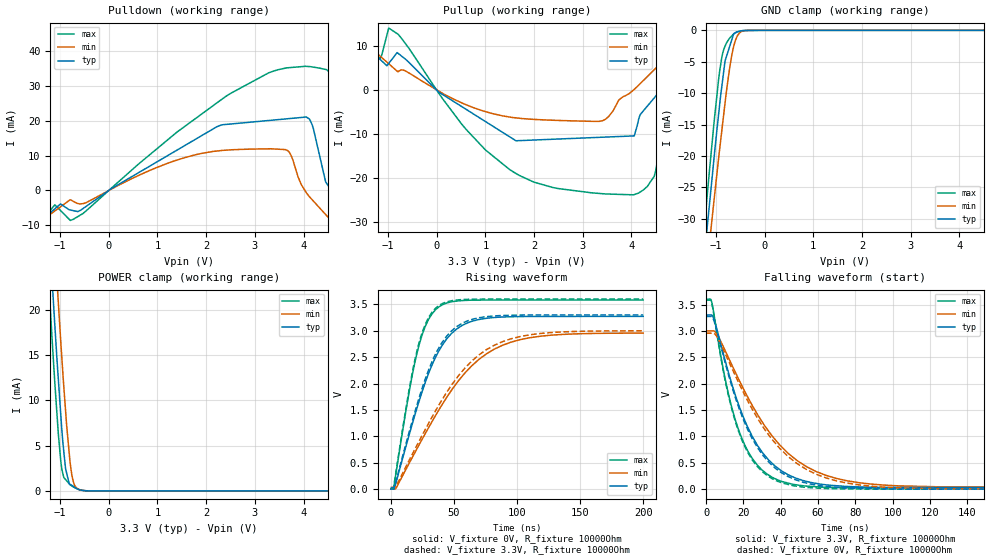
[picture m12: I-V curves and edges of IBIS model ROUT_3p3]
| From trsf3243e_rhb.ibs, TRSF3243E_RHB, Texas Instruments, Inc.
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[Model]   ROUT_3p3
Model_type   3-state
Polarity   Non-Inverting
Vmeas = 1.65
Vref = 0
Cref = 150pF
Rref = 3000
|variable   typ   min   max
C_comp   1.47pF   1.38pF   1.52pF
|C_pullup   1.38pF   1.27pF   1.45pF
|C_pulldown   1.80pF   1.75pF   1.86pF
[Voltage Range]   3.3   3   3.6
[Temperature Range]   27   110   -40
[Pullup Reference]   3.3   3   3.6
[Pulldown Reference]   0   0   0
[Power Clamp Reference]   3.3   3   3.6
[GND Clamp Reference]   0   0   0
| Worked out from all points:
|   slope of the pulldown table from 0 to 0.495 V, typ, clamps not added: 119 ohm
|   slope of the pullup table from 0 to 0.495 V, typ, clamps not added: 136 ohm
|   GND clamp passes 1 mA (typ) near -0.65 V on its own axis
|   POWER clamp passes 1 mA (typ) near -0.82 V on its own axis
|   falling waveform, V_fixture 3.3V, R_fixture 10000Ohm: 20-80 % time 21.7ns typ, 32.6ns min, 15.9ns max; typ from 3.3 V to 0.029 V
|   rising waveform, V_fixture 0V, R_fixture 10000Ohm: 20-80 % time 27.9ns typ, 48.7ns min, 17.3ns max; typ from 0 V to 3.27 V
|   rising waveform, V_fixture 3.3V, R_fixture 10000Ohm: 20-80 % time 27.3ns typ, 47.1ns min, 17ns max; typ from 0.029 V to 3.3 V
|   falling waveform, V_fixture 0V, R_fixture 10000Ohm: 20-80 % time 21.6ns typ, 32.1ns min, 15.9ns max; typ from 3.27 V to 0 V
[Pulldown]
|   Voltage   I(typ)   I(min)   I(max)
-3.3V     -787.1uA   -298.2uA   -879.3uA
-3.13V    -9.259mA   -8.11mA    -9.971mA
-788.7mV  -5.612mA   -2.71mA    -8.598mA
2.735V    19.39mA    11.81mA    29.64mA
4.042V    21.08mA    -312.1uA   35.66mA
4.523V    1.033mA    -7.969mA   33.99mA
4.925V    -7.207mA   -9.102mA   4.57mA
5.433V    -7.855mA   -9.28mA    -8.328mA
6.366V    -7.517mA   -9.606mA   -7.618mA
6.522V    -7.461mA   -6.718mA   -2.416mA
6.532V    24.7mA     -6.523mA   24.29mA
6.6V      231.2mA    268.8mA    195.7mA
[GND Clamp]
|   Voltage   I(typ)   I(min)   I(max)
-3.3V     -210.1mA   -202.3mA   -218.6mA
-1.348V   -45.17mA   -50.25mA   -41.18mA
-1.208V   -33.83mA   -39.74mA   -28.91mA
-1.175V   -31.12mA   -37.23mA   -26.05mA
-1.107V   -25.78mA   -32.11mA   -20.34mA
-942mV    -13.28mA   -20.29mA   -7.725mA
-879.8mV  -9.08mA    -16.12mA   -4.389mA
-811.2mV  -4.875mA   -11.57mA   -2.536mA
-686.3mV  -1.833mA   -4.566mA   -987.9uA
-577mV    -278.2uA   -1.197mA   -309.3uA
-315.2mV  -33.26uA   -7.242uA   -7.414uA
6.6V      0A         0A         0A
[Pullup]
|   Voltage   I(typ)   I(min)   I(max)
-3.3V     131.1uA    87.96uA    178.1uA
-3.13V    9.92mA     9.846mA    9.995mA
-1.163V   7.022mA    7.761mA    7.124mA
-984.1mV  6.064mA    6.007mA    14.15mA
1.499V    -10.66mA   -6.155mA   -18.13mA
3.404V    -10.76mA   -7.017mA   -23.64mA
4.042V    -10.46mA   18.97uA    -23.9mA
5.433V    5.648mA    6.097mA    6.407mA
6.366V    4.745mA    6.255mA    5.441mA
6.52V     4.596mA    3.972mA    5.281mA
6.532V    -24.61mA   3.786mA    -25.75mA
6.6V      -212.1mA   -227.5mA   -193.1mA
[POWER Clamp]
|   Voltage   I(typ)   I(min)   I(max)
-3.3V     230.9mA    239.1mA    225mA
-1.254V   31.57mA    40.43mA    25.24mA
-1.175V   24.31mA    33.19mA    17.85mA
-1.131V   20.41mA    29.18mA    13.95mA
-1.06V    14.27mA    22.94mA    8.245mA
-1.035V   12.33mA    20.8mA     6.311mA
-961.9mV  6.695mA    14.63mA    2.369mA
-887.3mV  2.484mA    8.947mA    1.267mA
-795.8mV  739.7uA    3.272mA    699uA
-760mV    616.4uA    1.855mA    553.7uA
-633.3mV  180.3uA    217uA      201.5uA
6.6V      0A         0A         0A
[Ramp]
R_load = 10000
|   typ   min   max
dV/dt_r   1.96363/2.79356e-08   1.77363/4.8671e-08   2.14915/1.72734e-08
dV/dt_f   1.96255/2.17589e-08   1.77823/3.26253e-08   2.14523/1.59509e-08
[Falling Waveform]
V_fixture = 3.3V
V_fixture_min = 3V
V_fixture_max = 3.6V
R_fixture = 10000Ohm
C_fixture = 0F
|   Time   V(typ)   V(min)   V(max)
0s        3.3V       3V         3.6V
3.021ns   3.301V     3.001V     3.545V
5.942ns   3.011V     2.932V     2.932V
11.03ns   2.329V     2.563V     1.951V
17.15ns   1.628V     2.106V     1.149V
24.77ns   996.4mV    1.584V     580.2mV
35.47ns   486.9mV    1.005V     223.6mV
53.77ns   147.3mV    427.5mV    58.24mV
75.54ns   51.26mV    158.8mV    29.98mV
200ns     29.08mV    36.28mV    24.61mV
[Rising Waveform]
V_fixture = 0V
V_fixture_min = 0V
V_fixture_max = 0V
R_fixture = 10000Ohm
C_fixture = 0F
|   Time   V(typ)   V(min)   V(max)
0s        -26.61nV   -137.3nV   -168.2nV
2.244ns   -755.5uV   -551.8uV   17.25mV
15.45ns   1.105V     530.2mV    1.962V
22.62ns   1.682V     849mV      2.75V
29.93ns   2.191V     1.164V     3.216V
38.16ns   2.62V      1.503V     3.453V
56.37ns   3.099V     2.132V     3.571V
88.29ns   3.26V      2.723V     3.582V
126.7ns   3.271V     2.916V     3.582V
200ns     3.273V     2.956V     3.582V
[Rising Waveform]
V_fixture = 3.3V
V_fixture_min = 3V
V_fixture_max = 3.6V
R_fixture = 10000Ohm
C_fixture = 0F
|   Time   V(typ)   V(min)   V(max)
0s        29.11mV    36.29mV    24.61mV
2.244ns   28.38mV    35.8mV     41.95mV
15.45ns   1.158V     588.3mV    2.01V
22.62ns   1.745V     918.4mV    2.795V
29.93ns   2.256V     1.246V     3.251V
38.16ns   2.679V     1.595V     3.479V
56.37ns   3.14V      2.227V     3.59V
88.29ns   3.289V     2.792V     3.6V
126.7ns   3.299V     2.965V     3.6V
200ns     3.3V       2.999V     3.6V
[Falling Waveform]
|Gnd
V_fixture = 0V
V_fixture_min = 0V
V_fixture_max = 0V
R_fixture = 10000Ohm
C_fixture = 0F
|   Time   V(typ)   V(min)   V(max)
0s        3.273V     2.957V     3.582V
3.021ns   3.272V     2.957V     3.524V
5.742ns   3.003V     2.895V     2.95V
11.03ns   2.287V     2.505V     1.922V
17.15ns   1.583V     2.04V      1.119V
24.77ns   953.9mV    1.513V     551.9mV
35.47ns   449.3mV    937.7mV    197.1mV
53.77ns   115.2mV    373.2mV    33.18mV
75.54ns   21.42mV    115.2mV    5.28mV
200ns     -27.36uV   -10.49uV   4.974uV
